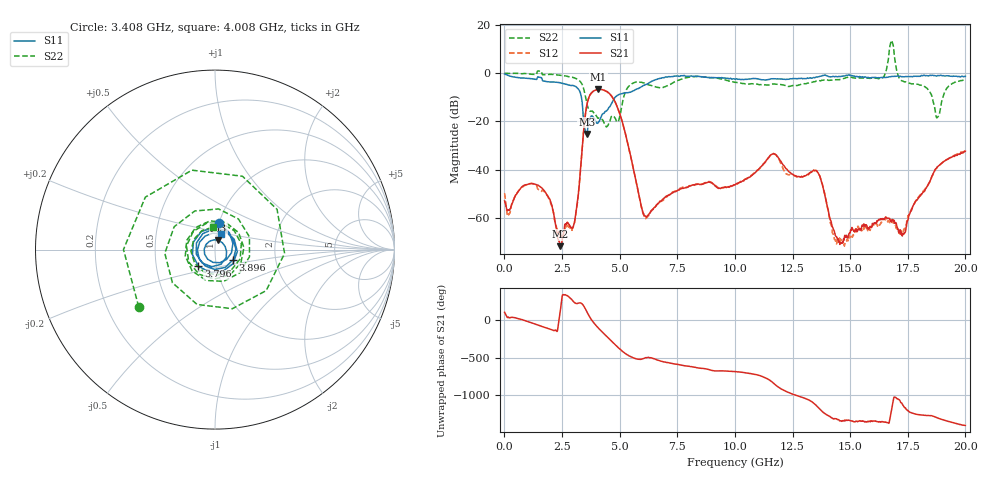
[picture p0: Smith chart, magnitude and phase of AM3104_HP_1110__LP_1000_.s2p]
!Created with skrf (http://scikit-rf.org).
# Hz S RI R 50.0
!freq ReS11 ImS11 ReS21 ImS21 ReS12 ImS12 ReS22 ImS22
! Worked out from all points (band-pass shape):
!   1601 points, 10 MHz to 20 GHz, reference 50 ohm
!   highest |S21| = -6.72 dB at 4.083 GHz (marker M1); lowest = -71.8 dB at 2.409 GHz (marker M2)
!   |S21| within 3 dB of the highest: 3.681 GHz to 4.667 GHz (985.7 MHz wide, 23.6 % of centre)
!   lowest |S11| = -25.2 dB at 3.571 GHz (marker M3), VSWR 1.12, Z = 51.7 + j5.33 ohm
!   |S11| at or under -10 dB: 3.342 GHz to 4.807 GHz (1.465 GHz wide, 36 % of centre)
!   |S22| runs from -22.3 to 13.5 dB; largest |S21 - S12| = 0.039
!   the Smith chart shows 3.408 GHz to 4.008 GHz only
!   S11 on the Smith chart (normalised r, x): 3.408 GHz: 1.00, +0.31; 3.796 GHz: 0.82, -0.15; 3.896 GHz: 1.22, -0.14; 4.008 GHz: 1.05, +0.18
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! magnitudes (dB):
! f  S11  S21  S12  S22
! 10 MHz  -0.4  -53.0  -49.8  -0.1
! 1.534 GHz  -1.7  -46.9  -48.6  0.9
! 2.409 GHz  -4.0  -71.8  -66.8  -0.9
! 2.996 GHz  -5.2  -63.4  -63.3  -1.8
! 3.346 GHz  -10.2  -34.8  -34.9  -4.2
! 3.408 GHz  -16.4  -27.3  -27.3  -5.5
! 3.571 GHz  -25.2  -13.5  -13.6  -12.3
! 3.796 GHz  -17.7  -8.0  -8.1  -15.7
! 3.896 GHz  -18.7  -7.3  -7.3  -16.5
! 4.008 GHz  -20.7  -6.9  -6.9  -18.0
! 4.083 GHz  -20.3  -6.7  -6.8  -18.6
! 4.958 GHz  -8.9  -15.4  -15.5  -19.7
! 6.057 GHz  -5.1  -58.8  -59.1  -4.1
! 6.682 GHz  -2.3  -53.9  -54.0  -6.0
! 10.01 GHz  -2.5  -46.4  -46.4  -3.8
! 11.64 GHz  -2.4  -33.6  -33.5  -4.5
! 13.34 GHz  -2.1  -40.9  -40.8  -3.8
! 14.4 GHz  -1.4  -67.9  -70.9  -2.7
! 16.68 GHz  -1.6  -60.2  -61.2  7.1
! 17.31 GHz  -1.5  -66.4  -65.3  -3.5
! 18.79 GHz  -1.0  -38.8  -39.0  -18.4
! 20 GHz  -1.4  -32.4  -32.3  -2.7
